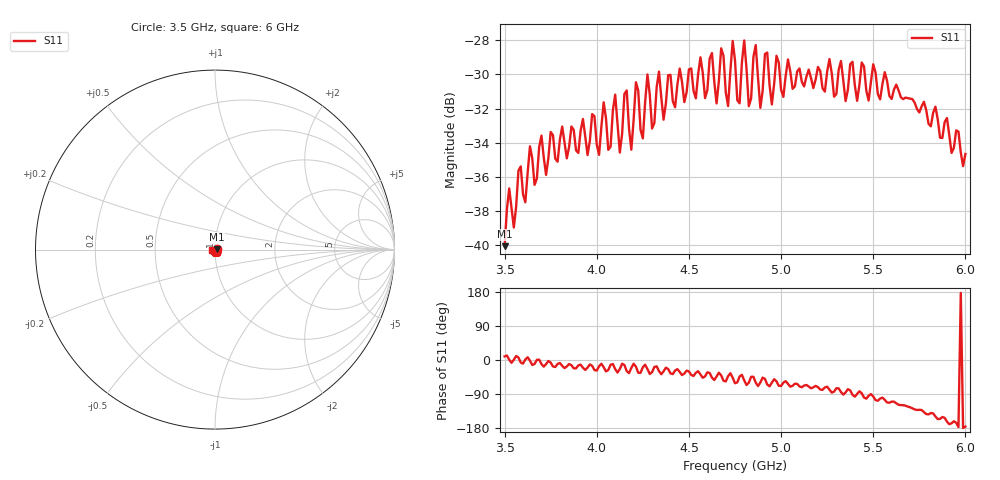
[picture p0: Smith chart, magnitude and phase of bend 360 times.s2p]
!  31/07/2025  14:40:18
! Ref Plane: 0.000 mm
# MHZ S MA R  50
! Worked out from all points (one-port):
!   201 points, 3.5 GHz to 6 GHz, reference 50 ohm
!   lowest |S11| = -40.1 dB at 3.5 GHz (marker M1), VSWR 1.02, Z = 51 + j0.167 ohm
!   |S11| at or under -10 dB: start of sweep to end of sweep
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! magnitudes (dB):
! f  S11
! 3.5 GHz  -40.1
! 3.525 GHz  -36.7
! 3.55 GHz  -39.0
! 3.638 GHz  -34.2
! 3.812 GHz  -33.1
! 4.013 GHz  -34.7
! 4.037 GHz  -31.6
! 4.062 GHz  -34.4
! 4.1 GHz  -31.2
! 4.125 GHz  -34.6
! 4.162 GHz  -30.9
! 4.188 GHz  -34.4
! 4.213 GHz  -30.5
! 4.25 GHz  -33.8
! 4.275 GHz  -30.0
! 4.3 GHz  -33.2
! 4.338 GHz  -29.8
! 4.362 GHz  -32.7
! 4.438 GHz  -30.6
! 4.625 GHz  -28.7
! 4.65 GHz  -31.7
! 4.675 GHz  -28.5
! 4.713 GHz  -31.9
! 4.75 GHz  -29.2
! 5.062 GHz  -30.8
! 5.375 GHz  -29.4
! 5.688 GHz  -31.4
! 6 GHz  -34.7
